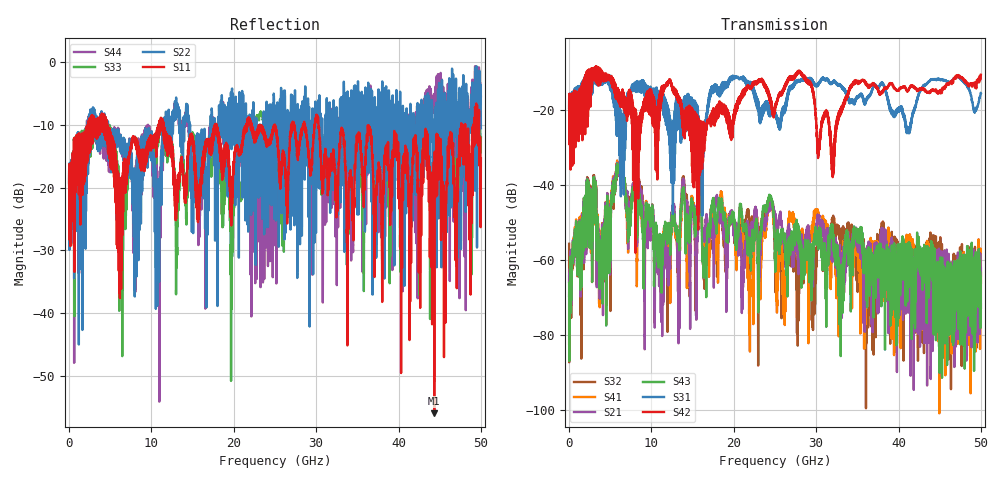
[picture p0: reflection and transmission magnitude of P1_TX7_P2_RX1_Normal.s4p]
!Keysight Technologies,N5225B,MY57041031,A.13.20.10
!Date: Friday, May 31, 2019 11:28:45
!Correction: S11(Full 4 Port(1,2,3,4))
!S12(Full 4 Port(1,2,3,4))
!S13(Full 4 Port(1,2,3,4))
!S14(Full 4 Port(1,2,3,4))
!S21(Full 4 Port(1,2,3,4))
!S22(Full 4 Port(1,2,3,4))
!S23(Full 4 Port(1,2,3,4))
!S24(Full 4 Port(1,2,3,4))
!S31(Full 4 Port(1,2,3,4))
!S32(Full 4 Port(1,2,3,4))
!S33(Full 4 Port(1,2,3,4))
!S34(Full 4 Port(1,2,3,4))
!S41(Full 4 Port(1,2,3,4))
!S42(Full 4 Port(1,2,3,4))
!S43(Full 4 Port(1,2,3,4))
!S44(Full 4 Port(1,2,3,4))
!S4P File: Measurements: <S11,S12,S13,S14>,
!<S21,S22,S23,S24>,
!<S31,S32,S33,S34>,
!<S41,S42,S43,S44>:
# Hz S  dB  R 50.0
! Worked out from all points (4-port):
!   5000 points, 10 MHz to 50 GHz, reference 50 ohm
!   strongest paths, dB at 10 MHz, 12.51 GHz, 25.01 GHz, 37.51 GHz, 50 GHz:
!     S42: -19.4, -14.2, -20.2, -14.7, -10.6
!     S31: -19.4, -38.9, -20.9, -14.0, -15.5
!     S43: -69.6, -48.4, -57.9, -58.0, -72.6
!     S21: -65.7, -47.6, -47.5, -64.1, -62.3
!     S41: -82.2, -48.8, -54.3, -66.0, -63.3
!     S32: -55.6, -48.1, -58.1, -57.4, -66.0
!   lowest |S11| = -56.0 dB at 44.34 GHz (marker M1), VSWR 1.00, Z = 49.8 - j0.0299 ohm
!   |S11| at or under -10 dB: 4.613 GHz to 10.86 GHz (6.246 GHz wide, 80.7 % of centre); 11.46 GHz to 17.73 GHz (6.278 GHz wide, 43 % of centre); 30.28 GHz to 47.6 GHz (17.32 GHz wide, 44.5 % of centre)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
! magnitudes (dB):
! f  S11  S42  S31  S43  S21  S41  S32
! 10 MHz  -19.2  -19.4  -19.4  -69.6  -65.7  -82.2  -55.6
! 5.98 GHz  -20.5  -14.6  -19.8  -35.4  -35.5  -34.8  -36.2
! 11.28 GHz  -10.2  -13.6  -17.8  -64.7  -60.7  -63.3  -60.4
! 13.88 GHz  -18.6  -21.3  -19.1  -41.0  -38.7  -40.6  -37.8
! 16.44 GHz  -13.9  -24.3  -25.2  -57.1  -54.2  -55.7  -67.6
! 44.34 GHz  -56.0  -15.0  -11.8  -62.8  -60.2  -67.1  -63.5
! 50 GHz  -15.3  -10.6  -15.5  -72.6  -62.3  -63.3  -66.0
